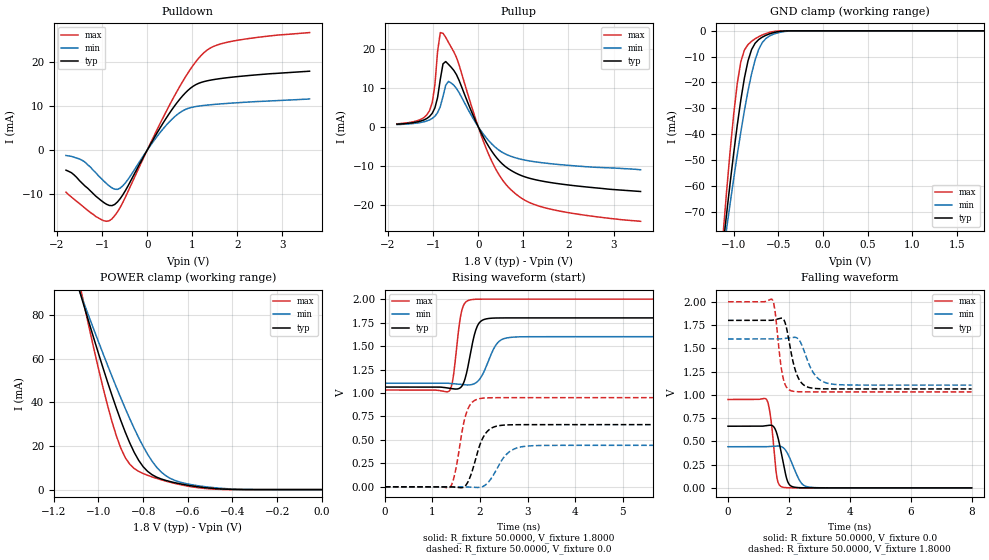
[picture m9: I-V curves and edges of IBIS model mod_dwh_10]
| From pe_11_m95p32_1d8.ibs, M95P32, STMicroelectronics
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|   Model mod_dwh_10
[Model]   mod_dwh_10
Model_type I/O
Polarity   Non-Inverting
Enable   Active-High
Vinl   =   0.540V
Vinh   =   1.260V
Vmeas  =   0.900V
Cref   =   30.0pF
C_comp   1.630pF   1.607pF   1.683pF
[Model Spec]
Vinl   0.540V  0.480V  0.600V  | <- for Vcc = 1.8V, 1.6V, 2.0V
Vinh   1.260V  1.120V  1.400V  | <- for Vcc = 1.8V, 1.6V, 2.0V
Vmeas  0.900V  0.800V  1.000V  | <- for Vcc = 1.8V, 1.6V, 2.0V
[Temperature Range]  25.0000   0.1050k   -40.0000
[Voltage Range]   1.8000V   1.6000V   2.0000V
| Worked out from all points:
|   slope of the pulldown table from 0 to 0.27 V, typ, clamps not added: 56.7 ohm
|   slope of the pullup table from 0 to 0.27 V, typ, clamps not added: 46.9 ohm
|   GND clamp passes 1 mA (typ) near -0.58 V on its own axis
|   POWER clamp passes 1 mA (typ) near -0.53 V on its own axis
|   rising waveform, R_fixture 50.0000, V_fixture 1.8000: 20-80 % time 184ps typ, 261ps min, 136ps max; typ from 1.06 V to 1.8 V
|   rising waveform, R_fixture 50.0000, V_fixture 0.0: 20-80 % time 257ps typ, 337ps min, 204ps max; typ from 0 V to 0.662 V
|   falling waveform, R_fixture 50.0000, V_fixture 0.0: 20-80 % time 252ps typ, 354ps min, 173ps max; typ from 0.662 V to 0 V
|   falling waveform, R_fixture 50.0000, V_fixture 1.8000: 20-80 % time 306ps typ, 412ps min, 204ps max; typ from 1.8 V to 1.06 V
[Pulldown]
|Voltage   I(typ)   I(min)   I(max)
-1.8V     -4.52mA    -1.2mA     -9.5mA
-1.38V    -8.1mA     -2.7mA     -13.1mA
-1.02V    -11.4mA    -6.38mA    -15.69mA
-840mV    -12.5mA    -8.1mA     -15.97mA
-660mV    -11.73mA   -8.87mA    -13.97mA
-540mV    -10.1mA    -8.054mA   -11.83mA
240mV     4.255mA    3.386mA    5.068mA
660mV     10.73mA    8.002mA    13.3mA
960mV     14.02mA    9.615mA    18.34mA
1.26V     15.51mA    10.12mA    22.07mA
1.92V     16.55mA    10.68mA    24.71mA
3.6V      17.86mA    11.6mA     26.6mA
[Pullup]
|Voltage   I(typ)   I(min)   I(max)
-1.8V     640uA      530uA      730uA
-1.08V    2.616mA    1.736mA    4.081mA
-960mV    4.827mA    2.686mA    10.73mA
-900mV    7.507mA    3.603mA    19.37mA
-840mV    12.2mA     5.175mA    24.19mA
-780mV    16.15mA    7.795mA    23.99mA
-660mV    16.03mA    11.63mA    21.69mA
-540mV    14.45mA    10.66mA    19.23mA
180mV     -4.048mA   -2.871mA   -5.668mA
720mV     -11.18mA   -7.584mA   -16.12mA
1.56V     -14.27mA   -9.451mA   -21.07mA
3.6V      -16.65mA   -11.06mA   -24.31mA
[GND_clamp]
|Voltage   I(typ)   I(min)   I(max)
-1.8V     -319.7mA   -274.4mA   -407.3mA
-1.12V    -83.64mA   -87.01mA   -79.32mA
-1.08V    -71.08mA   -76.85mA   -62.45mA
-1V       -47.38mA   -57.28mA   -32.33mA
-960mV    -36.55mA   -47.99mA   -20.38mA
-920mV    -26.73mA   -39.15mA   -11.92mA
-840mV    -11.67mA   -23.32mA   -5.34mA
-760mV    -4.801mA   -11.23mA   -3.081mA
-720mV    -3.384mA   -7.183mA   -2.279mA
-640mV    -1.748mA   -2.99mA    -1.048mA
-440mV    -85.93uA   -314uA     -8.035uA
1.8V      367pA      1.678uA    95.55pA
[POWER_clamp]
|Voltage   I(typ)   I(min)   I(max)
-1.8V     354.3mA    299.2mA    462.7mA
-1.08V    89.41mA    89.52mA    92.12mA
-1.06V    82.53mA    84.01mA    82.65mA
-980mV    55.86mA    62.44mA    46.9mA
-920mV    37.35mA    46.96mA    24.63mA
-880mV    26.31mA    37.17mA    14.66mA
-840mV    17.07mA    28.03mA    9.669mA
-800mV    10.51mA    19.82mA    7.37mA
-740mV    5.731mA    10.32mA    5.151mA
-640mV    2.77mA     3.598mA    2.408mA
-420mV    154.7uA    391.9uA    29.01uA
0V        367pA      12.25nA    169pA
[Ramp]
| variable   typ   min   max
dV/dt_r   0.3975/0.3147n   0.2652/0.4704n   0.5700/0.2297n
dV/dt_f   0.4421/0.4092n   0.2972/0.5944n   0.5812/0.2321n
R_load = 50.0000
[Rising Waveform]
R_fixture= 50.0000
V_fixture= 1.8000
V_fixture_min= 1.6000
V_fixture_max= 2.0000
|time   V(typ)   V(min)   V(max)
0s        1.063V     1.104V     1.031V
1.352ns   1.051V     1.103V     1.02V
1.432ns   1.044V     1.099V     1.149V
1.608ns   1.066V     1.09V      1.857V
1.8ns     1.421V     1.087V     1.993V
1.896ns   1.645V     1.103V     1.998V
2.008ns   1.76V      1.157V     2V
2.328ns   1.799V     1.505V     2V
2.584ns   1.8V       1.588V     2V
8ns       1.8V       1.6V       2V
[Rising Waveform]
R_fixture= 50.0000
V_fixture= 0.0
V_fixture_min= 0.0
V_fixture_max= 0.0
|time   V(typ)   V(min)   V(max)
0s        4.25nV     554.9nV    665.8pV
1.376ns   -350.7uV   433.2uV    -1.737mV
1.472ns   -3.381mV   404.3uV    138.7mV
1.712ns   22.35mV    -1.472mV   783.9mV
1.824ns   148.6mV    -4.251mV   894.1mV
1.984ns   426.9mV    -6.696mV   938.9mV
2.256ns   629.4mV    103.8mV    949.3mV
2.56ns    659.3mV    347.5mV    950mV
2.896ns   662.2mV    428.3mV    950.1mV
8ns       662.5mV    442mV      950.1mV
[Falling Waveform]
R_fixture= 50.0000
V_fixture= 0.0
V_fixture_min= 0.0
V_fixture_max= 0.0
|time   V(typ)   V(min)   V(max)
0s        662.5mV    442mV      950.1mV
1.272ns   669.1mV    442.6mV    945.6mV
1.4ns     673.3mV    445.6mV    757.4mV
1.608ns   578.9mV    450.3mV    107.7mV
1.768ns   346.7mV    441mV      10.42mV
1.912ns   116.8mV    394.3mV    2.004mV
2.008ns   37.96mV    335mV      706.2uV
2.36ns    1.729mV    74.11mV    19.84uV
2.616ns   240.4uV    11.16mV    3.293uV
8ns       610nV      1.031uV    778.7nV
[Falling Waveform]
R_fixture= 50.0000
V_fixture= 1.8000
V_fixture_min= 1.6000
V_fixture_max= 2.0000
|time   V(typ)   V(min)   V(max)
0s        1.8V       1.6V       2V
1.472ns   1.803V     1.6V       2.014V
1.552ns   1.808V     1.6V       1.881V
1.792ns   1.822V     1.603V     1.208V
2.064ns   1.468V     1.614V     1.045V
2.24ns    1.235V     1.615V     1.034V
2.432ns   1.121V     1.529V     1.032V
2.8ns     1.07V      1.238V     1.031V
3.248ns   1.064V     1.126V     1.031V
8ns       1.063V     1.105V     1.031V
